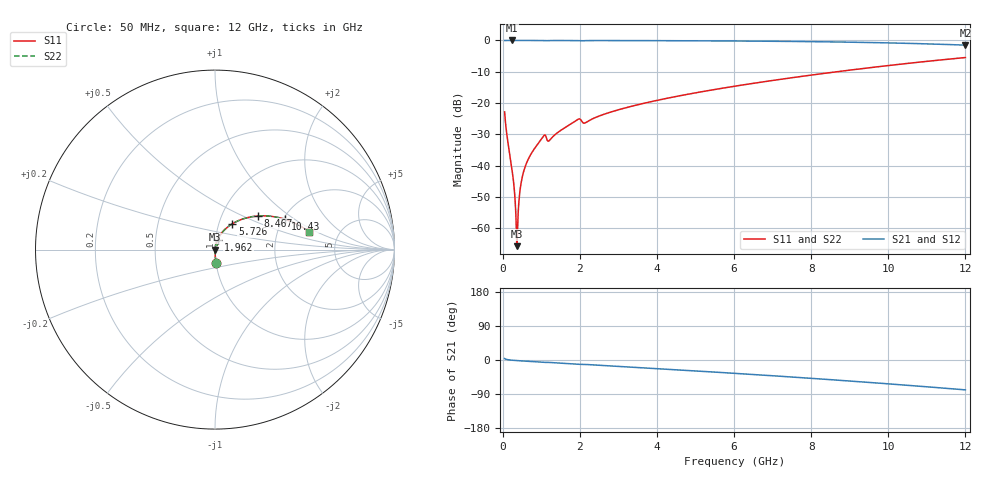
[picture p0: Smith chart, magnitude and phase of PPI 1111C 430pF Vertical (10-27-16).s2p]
# GHz S MA R 50
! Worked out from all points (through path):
!   1601 points, 50 MHz to 12 GHz, reference 50 ohm
!   highest |S21| = 0.00 dB at 244.2 MHz (marker M1); lowest = -1.5 dB at 12 GHz (marker M2)
!   group delay of S21, straight-line fit = 18.1 ps
!   lowest |S11| = -65.7 dB at 371.2 MHz (marker M3), VSWR 1.00, Z = 50.1 + j0.00723 ohm
!   |S11| at or under -10 dB: start of sweep to 8.666 GHz
!   |S22| runs from -65.7 to -5.5 dB; largest |S21 - S12| = 0
!   S11 on the Smith chart (normalised r, x): 50 MHz: 1.00, -0.15; 1.962 GHz: 1.03, +0.11; 5.726 GHz: 1.16, +0.34; 8.467 GHz: 1.48, +0.61; 10.43 GHz: 2.05, +0.84; 12 GHz: 3.02, +0.84
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0.05  0.07241 -85.9  0.9971 3.9  0.9971 3.9  0.07241 -85.9
0.2441875  0.008561 -87.6  0.9995 -0.5  0.9995 -0.5  0.008561 -87.6
0.2815313  0.005547 -86.1  0.9995 -0.9  0.9995 -0.9  0.005547 -86.1
0.3263437  0.002552 -80.3  0.9995 -1.2  0.9995 -1.2  0.002552 -80.3
0.3711563  0.0005176 8.0  0.9995 -1.5  0.9995 -1.5  0.0005176 8.0
0.4085  0.00209 73.5  0.9994 -1.8  0.9994 -1.8  0.00209 73.5
0.46825  0.004859 81.1  0.9994 -2.2  0.9994 -2.2  0.004859 81.1
0.528  0.007409 82.8  0.9993 -2.6  0.9993 -2.6  0.007409 82.8
0.6325625  0.01153 83.4  0.9992 -3.3  0.9992 -3.3  0.01153 83.4
0.7744688  0.01683 83.2  0.999 -4.2  0.999 -4.2  0.01683 83.2
1.058281  0.0297 75.4  0.9951 -6.1  0.9951 -6.1  0.0297 75.4
1.215125  0.02539 74.0  0.9954 -6.5  0.9954 -6.5  0.02539 74.0
1.962  0.05537 71.0  0.991 -11.3  0.991 -11.3  0.05537 71.0
2.044156  0.05197 63.7  0.9852 -11.4  0.9852 -11.4  0.05197 63.7
4.038312  0.1115 66.1  0.9919 -23.0  0.9919 -23.0  0.1115 66.1
5.72625  0.1738 56.0  0.9825 -33.3  0.9825 -33.3  0.1738 56.0
6.025  0.1861 54.2  0.9802 -35.2  0.9802 -35.2  0.1861 54.2
8.019156  0.2807 41.0  0.9569 -48.5  0.9569 -48.5  0.2807 41.0
8.467281  0.3051 37.9  0.9492 -51.6  0.9492 -51.6  0.3051 37.9
10.01331  0.398 26.6  0.9137 -63.0  0.9137 -63.0  0.398 26.6
10.43156  0.4253 23.3  0.9013 -66.2  0.9013 -66.2  0.4253 23.3
12  0.5333 10.8  0.8415 -78.8  0.8415 -78.8  0.5333 10.8
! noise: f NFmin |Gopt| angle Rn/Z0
0.05  0.0003433  0.8556  0.2587  0.0005079
1.372  0.004813  0.7361  5.611  0.003636
2.701  0.006653  0.6457  10.79  0.003527
4.031  0.008125  0.5865  15.64  0.003527
5.36  0.01001  0.5655  20.33  0.004035
6.682  0.01198  0.5571  24.82  0.004644
8.012  0.01408  0.5573  29.16  0.005372
9.341  0.01637  0.5646  33.36  0.006258
10.67  0.01892  0.578  37.45  0.007366
12  0.02183  0.5969  41.48  0.008785
